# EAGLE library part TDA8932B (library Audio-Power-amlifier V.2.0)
The TDA8932B is a high efficiency class-D amplifier with low power dissipation. The continuous time output power is 2 ´ 15 W in stereo half-bridge application (RL = 4 W) or 1 ´ 30 W in mono full-bridge application (RL = 8 W). Due to the low power dissipation the device can be used without any external heat sink when playing music. Due to the implementation of thermal foldback, even for high supply voltages and/or lower load impedances, the device continues to operate with considerable music output power without the need for an external heat sink.
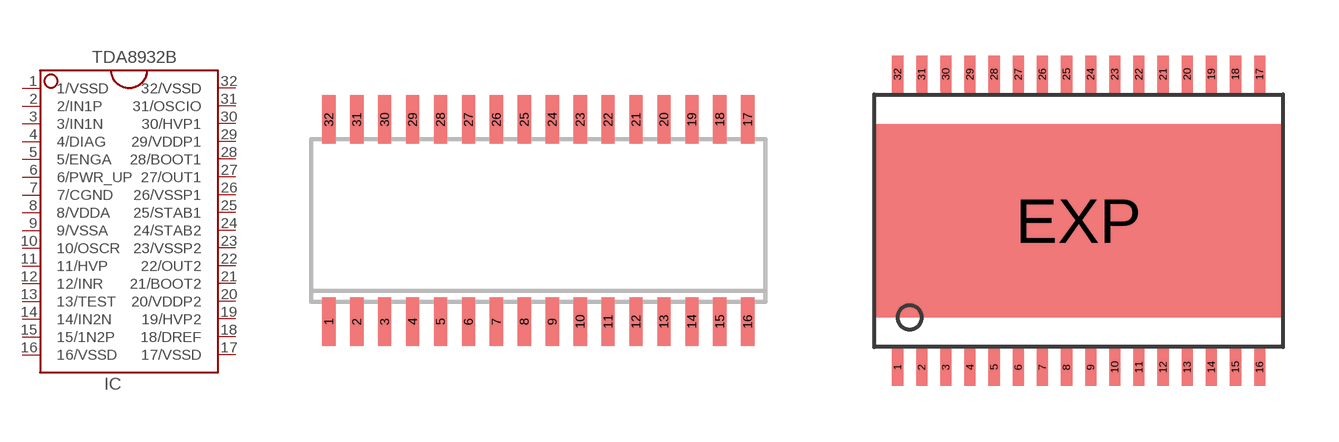
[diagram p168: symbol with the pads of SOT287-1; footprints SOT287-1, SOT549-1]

Designator prefix IC

## TDA8932BTDA8932BT  [SOT287-1]
1  1/VSSD  pwr
2  2/IN1P  in
3  3/IN1N  in
4  4/DIAG  out
5  5/ENGA  in
6  6/PWR_UP  in
7  7/CGND  pwr
8  8/VDDA  pwr
9  9/VSSA  pwr
10  10/OSCR  in
11  11/HVP
12  12/INR  in
13  13/TEST  in
14  14/IN2N  in
15  15/1N2P  in
16  16/VSSD  pwr
17  17/VSSD  pwr
18  18/DREF  in
19  19/HVP2  out
20  20/VDDP2  pwr
21  21/BOOT2
22  22/OUT2  out
23  23/VSSP2  pwr
24  24/STAB2  pwr
25  25/STAB1  pwr
26  26/VSSP1  pwr
27  27/OUT1  out
28  28/BOOT1
29  29/VDDP1  pwr
30  30/HVP1  out
31  31/OSCIO  in
32  32/VSSD  pwr

## TDA8932BTDA8932BTW  [SOT549-1]
Pads as for SOT287-1

## Footprint SOT287-1 (pad centres in mm)
SMALL OUTLINE INTEGRATED CIRCUIT wide body 7.5 mm/JEDEC MO-119AB
smd 0.6 x 2.2: 1 -9.525,-4.6; 2 -8.255,-4.6; 3 -6.985,-4.6; 4 -5.715,-4.6; 5 -4.445,-4.6; 6 -3.175,-4.6; 7 -1.905,-4.6; 8 -0.635,-4.6; 9 0.635,-4.6; 10 1.905,-4.6; 11 3.175,-4.6; 12 4.445,-4.6; 13 5.715,-4.6; 14 6.985,-4.6; 15 8.255,-4.6; 16 9.525,-4.6; 17 9.525,4.6; 18 8.255,4.6; 19 6.985,4.6; 20 5.715,4.6; 21 4.445,4.6; 22 3.175,4.6; 23 1.905,4.6; 24 0.635,4.6; 25 -0.635,4.6; 26 -1.905,4.6; 27 -3.175,4.6; 28 -4.445,4.6; 29 -5.715,4.6; 30 -6.985,4.6; 31 -8.255,4.6; 32 -9.525,4.6

## Footprint SOT549-1 (pad centres in mm)
PowerPAD(TM) PLASTIC SMALL-OUTLINE PACKAGE DAP (R-PDSO-G**)
smd 0.3 x 1: 1 -4.875,-3.95; 2 -4.225,-3.95; 3 -3.575,-3.95; 4 -2.925,-3.95; 5 -2.275,-3.95; 6 -1.625,-3.95; 7 -0.975,-3.95; 8 -0.325,-3.95; 9 0.325,-3.95; 10 0.975,-3.95; 11 1.625,-3.95; 12 2.275,-3.95; 13 2.925,-3.95; 14 3.575,-3.95; 15 4.225,-3.95; 16 4.875,-3.95; 17 4.875,3.95; 18 4.225,3.95; 19 3.575,3.95; 20 2.925,3.95; 21 2.275,3.95; 22 1.625,3.95; 23 0.975,3.95; 24 0.325,3.95; 25 -0.325,3.95; 26 -0.975,3.95; 27 -1.625,3.95; 28 -2.275,3.95; 29 -2.925,3.95; 30 -3.575,3.95; 31 -4.225,3.95; 32 -4.875,3.95
smd 11 x 5.2: EXP 0,0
